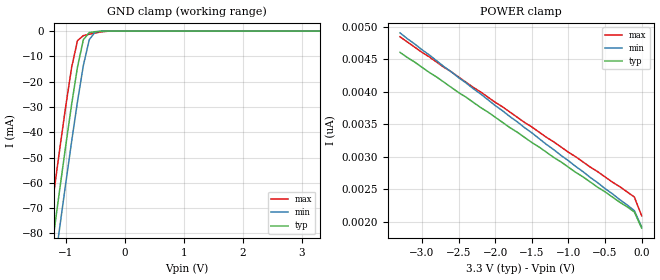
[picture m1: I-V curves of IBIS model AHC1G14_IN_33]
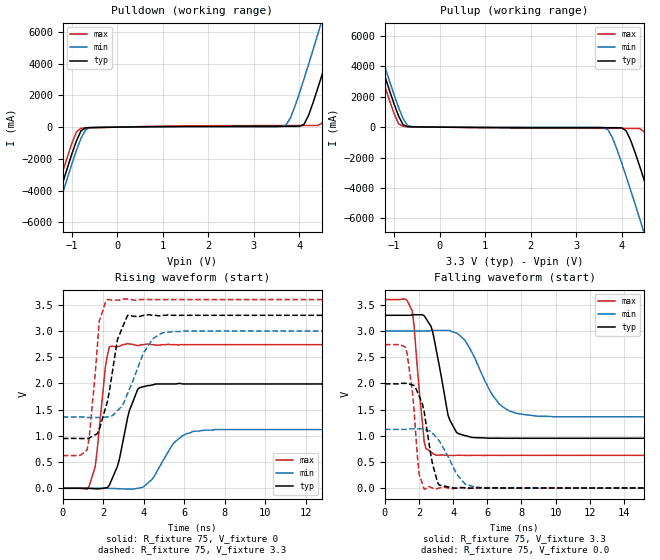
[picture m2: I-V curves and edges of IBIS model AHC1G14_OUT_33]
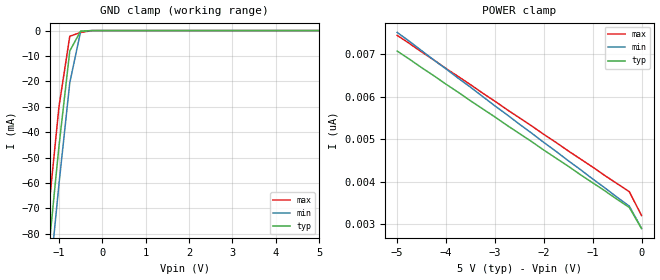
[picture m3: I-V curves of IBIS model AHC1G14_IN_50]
| TEXAS INSTRUMENTS INCORPORATED
| Standard Linear and Logic Group
| IBIS Model of SN74AHC1G14
| SINGLE SCHMITT-TRIGGER INVERTER
| SOT 5-pin (DCK) and SOT 5-pin (DBV) Package
[IBIS Ver]   3.2
[Comment Char]  |_char
[File Name]   ahc1g14.ibs
[File Rev]   2.0 J_die
[Date]   May 24, 2000
[Source]   Data created from HSPICE simulations at TI-SLL.
[Notes]   The following is an IBIS list for the AHC1G14.
|   Please contact sllibis@ti.com with questions and
|   comments concerning SLL IBIS models.
[Disclaimer] Property of Texas Instruments Incorporated.  Unauthorized
   reproduction and/or distribution is strictly prohibited.
   This product is protected under copyright law.
   Created 2000, (C) Copyright 2000, Texas Instruments Inc.,
   All Rights Reserved.
   UNLESS THERE IS A SIGNED, WRITTEN AGREEMENT TO THE
   CONTRARY, TEXAS INSTRUMENTS () IS PROVIDING THE IBIS
   MODELS  AND WITHOUT ANY WARRANTY, EXPRESSED OR
   IMPLIED.  TI assumes no liability for:
   1) the accuracy of the IBIS models provided to your
   company;
   2) the proper functioning of these IBIS Models in your
   design or for any resulting applications; or
   3) infringement of patents, copyrights or intellectual
   property rights resulting from your use of these IBIS
   models.
   TI provides IBIS Models as a service to our customers.
   You and your company shall not distribute, sell or give
   these models to anyone else without prior written
   permission from TI.
   TI reserves the right to make changes to our products or
   to discontinue any semiconductor product or service
   without notice, and advises our customers to obtain the
   latest version of relevant information to verify, before
   placing orders, that the information being relied on is
   current.
   Please be aware that your receipt and use of the IBIS
   information provided shall serve as acceptance of these
   terms and conditions.  If you do not accept these terms,
   you should return or destroy the IBIS models and any
   other accompanying information immediately.
|   Component AHC1G14_DCK
[Component]   AHC1G14_DCK
[Manufacturer]  Texas Instruments, Inc.
[Package]
|   typ   min   max
R_pkg   0.020   0.017   0.025
L_pkg   0.998nH   0.881nH   1.069nH
C_pkg   0.146pF   0.118pF   0.205pF
[Pin]   signal_name   model_name   R_pin   L_pin   C_pin
1   NC   NC   0.019   1.069nH   0.162pF
2   A   AHC1G14_IN   0.018   0.881nH   0.121pF
3   GND   GND   0.017   1.031nH   0.205pF
4   Y   AHC1G14_OUT   0.020   0.960nH   0.124pF
5   VCC   POWER   0.025   1.049nH   0.118pF
|   Component AHC1G14_DBV
[Component]   AHC1G14_DBV
[Manufacturer]  Texas Instruments, Inc.
[Package]
|   typ   min   max
R_pkg   0.025   0.021   0.029
L_pkg   1.529nH   1.312nH   1.906nH
C_pkg   0.156pF   0.110pF   0.240pF
[Pin]   signal_name   model_name   R_pin   L_pin   C_pin
1   NC   NC   0.021   1.511nH   0.144pF
2   A   AHC1G14_IN   0.023   1.312nH   0.138pF
3   GND   GND   0.029   1.906nH   0.240pF
4   Y   AHC1G14_OUT   0.026   1.541nH   0.150pF
5   VCC   POWER   0.025   1.374nH   0.110pF
[Model Selector]   AHC1G14_IN
AHC1G14_IN_33   3.3-V Vcc Input Model
AHC1G14_IN_50   5.0-V Vcc Input Model
[Model Selector]   AHC1G14_OUT
AHC1G14_OUT_33   3.3-V Vcc Output Model
AHC1G14_OUT_50   5.0-V Vcc Output Model
| Models and submodels in the file (4): AHC1G14_IN_33 (Input), AHC1G14_OUT_33 (Output), AHC1G14_IN_50 (Input), AHC1G14_OUT_50 (Output)
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|   Model AHC1G14_IN_33
[Model]   AHC1G14_IN_33
Model_type  Input
Polarity   Inverting
Vinl = 0.99
Vinh = 2.31
| variable   typ   min   max
C_comp   1.27pf   0.95pf   1.59pf
[Temperature Range]   25   85   -40
[Voltage Range]   3.3   3.0   3.6
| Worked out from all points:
|   GND clamp passes 1 mA (typ) near -0.61 V on its own axis
[GND Clamp]
|   Voltage   I(typ)   I(min)   I(max)
-3.3V     -460mA     -475mA     -445mA
-1.3V     -97.5mA    -113mA     -81.5mA
-1.2V     -79.9mA    -95mA      -63.9mA
-1.1V     -62.6mA    -77.6mA    -46.7mA
-1V       -45.6mA    -60.5mA    -30mA
-900mV    -29.2mA    -43.9mA    -14.6mA
-800mV    -14.3mA    -28mA      -3.81mA
-700mV    -3.42mA    -13.6mA    -1.78mA
-600mV    -581uA     -3.4mA     -1.25mA
-500mV    -233uA     -353uA     -759uA
-400mV    -58.1uA    -21.9uA    -324uA
3.3V      1.9nA      2.34nA     1.69nA
[POWER Clamp]
|   Voltage   I(typ)   I(min)   I(max)
-3.3V     4.61nA     4.91nA     4.85nA
-3V       4.38nA     4.65nA     4.61nA
-100mV    2.15nA     2.17nA     2.38nA
0V        1.9nA      1.92nA     2.09nA
|   Model AHC1G14_OUT_33
[Model]   AHC1G14_OUT_33
Model_type  Output
Polarity   Inverting
Vmeas = 1.65v
Cref = 15pf
| variable   typ   min   max
C_comp   3.12pf   2.34pf   3.90pf
[Temperature Range]   25   85   -40
[Voltage Range]   3.3   3.0   3.6
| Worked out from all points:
|   slope of the pulldown table from 0 to 0.495 V, typ, clamps not added: 26.1 ohm
|   slope of the pullup table from 0 to 0.495 V, typ, clamps not added: 40.3 ohm
|   rising waveform, R_fixture 75, V_fixture 0: 20-80 % time 728ps typ, 1.06ns min, 428ps max; typ from 0 V to 1.99 V
|   falling waveform, R_fixture 75, V_fixture 3.3: 20-80 % time 790ps typ, 1.54ns min, 473ps max; typ from 3.3 V to 0.95 V
|   rising waveform, R_fixture 75, V_fixture 3.3: 20-80 % time 673ps typ, 1.07ns min, 398ps max; typ from 0.95 V to 3.3 V
|   falling waveform, R_fixture 75, V_fixture 0.0: 20-80 % time 635ps typ, 1.12ns min, 459ps max; typ from 1.99 V to 0 V
[Pulldown]
|   Voltage   I(typ)   I(min)   I(max)
-3.3V     -24A       -24.6A     -23.4A
-1.6V     -7.31A     -7.95A     -6.63A
-1.5V     -6.34A     -6.99A     -5.66A
-1V       -1.69A     -2.33A     -1.02A
-800mV    -234mA     -703mA     -70.7mA
-600mV    -28.4mA    -27.3mA    -48.1mA
3.7V      47.1mA     113mA      100mA
4.1V      173mA      3.03A      101mA
4.4V      2.42A      5.83A      105mA
4.8V      6.17A      9.67A      2.68A
5.2V      10A        13.6A      6.5A
6.6V      23.8A      27.4A      20.3A
[Pullup]
|   Voltage   I(typ)   I(min)   I(max)
-3.3V     23.8A      24.4A      23.2A
-1.6V     7.13A      7.74A      6.5A
-1.5V     6.17A      6.78A      5.53A
-1V       1.53A      2.14A      903mA
-800mV    158mA      559mA      49mA
-600mV    19.5mA     16.8mA     33.4mA
3.7V      -35.9mA    -168mA     -78.9mA
4.1V      -236mA     -3.23A     -83.5mA
4.4V      -2.58A     -6.03A     -95.5mA
4.8V      -6.34A     -9.88A     -2.81A
5.2V      -10.2A     -13.8A     -6.63A
6.6V      -24A       -27.6A     -20.4A
[Ramp]
| variable   typ   min   max
dV/dt_r   1.20E+00/6.26E-10   6.82E-01/1.06E-09   1.65E+00/3.52E-10
dV/dt_f   1.42E+00/7.56E-10   9.96E-01/1.51E-09   1.80E+00/4.08E-10
R_load = 75
[Rising Waveform]
R_fixture = 75
V_fixture = 0
|   Time   V(typ)   V(min)   V(max)
0s        0V         0V         0V
1.3ns     -1.93mV    414uV      41.8mV
1.6ns     -9.28mV    217uV      407mV
2.1ns     6.59mV     -1.35mV    2.31V
2.3ns     60.1mV     -2.76mV    2.7V
2.8ns     564mV      -8.9mV     2.71V
3.3ns     1.5V       -15.8mV    2.75V
4.2ns     1.96V      100mV      2.75V
6.5ns     1.99V      1.09V      2.74V
25ns      1.99V      1.12V      2.74V
[Falling Waveform]
R_fixture = 75
V_fixture = 3.3
V_fixture_min = 3.0
V_fixture_max = 3.6
|   Time   V(typ)   V(min)   V(max)
0s        3.3V       3V         3.6V
1.2ns     3.3V       3V         3.61V
1.6ns     3.31V      3V         3.38V
2.3ns     3.29V      3V         889mV
3ns       2.65V      3.01V      627mV
3.8ns     1.3V       3.01V      621mV
5.1ns     966mV      2.59V      624mV
6.7ns     952mV      1.6V       624mV
7.8ns     950mV      1.42V      623mV
25ns      950mV      1.36V      624mV
[Rising Waveform]
R_fixture = 75
V_fixture = 3.3
V_fixture_min = 3.0
V_fixture_max = 3.6
|   Time   V(typ)   V(min)   V(max)
0s        950mV      1.36V      624mV
1.2ns     948mV      1.35V      731mV
1.4ns     979mV      1.35V      1.36V
1.8ns     1.12V      1.35V      3.19V
2.2ns     1.65V      1.36V      3.6V
2.7ns     2.84V      1.48V      3.59V
3.2ns     3.3V       1.81V      3.61V
4ns       3.3V       2.59V      3.6V
5.1ns     3.3V       2.98V      3.6V
25ns      3.3V       3V         3.6V
[Falling Waveform]
R_fixture = 75
V_fixture = 0.0
|   Time   V(typ)   V(min)   V(max)
0s        1.99V      1.12V      2.74V
1.3ns     2V         1.12V      2.57V
1.6ns     1.97V      1.13V      1.87V
2ns       1.76V      1.13V      273mV
2.3ns     1.46V      1.12V      -22mV
2.7ns     611mV      1.08V      11.4mV
3.1ns     91.5mV     930mV      -7.42mV
4ns       1.33mV     401mV      -10.9mV
5.7ns     1.89mV     8.33mV     -144uV
25ns      0V         0V         0V
|   Model AHC1G14_IN_50
[Model]   AHC1G14_IN_50
Model_type  Input
Polarity   Inverting
Vinl = 1.5
Vinh = 3.5
| variable   typ   min   max
C_comp   1.27pf   0.95pf   1.59pf
[Temperature Range]   25   85   -40
[Voltage Range]   5.0   4.5   5.5
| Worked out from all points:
|   GND clamp passes 1 mA (typ) near -0.52 V on its own axis
[GND Clamp]
|   Voltage   I(typ)   I(min)   I(max)
-5V       -773mA     -786mA     -758mA
-1.5V     -133mA     -148mA     -117mA
-1.25V    -88.7mA    -104mA     -72.7mA
-1V       -45.6mA    -60.5mA    -30mA
-750mV    -7.99mA    -20.5mA    -2.23mA
-500mV    -233uA     -353uA     -759uA
-250mV    -2.63nA    -182nA     -26.9uA
5V        2.9nA      3.64nA     2.54nA
[POWER Clamp]
|   Voltage   I(typ)   I(min)   I(max)
-5V       7.08nA     7.52nA     7.45nA
-1.5V     4.37nA     4.5nA      4.73nA
-250mV    3.4nA      3.43nA     3.77nA
0V        2.9nA      2.91nA     3.21nA
